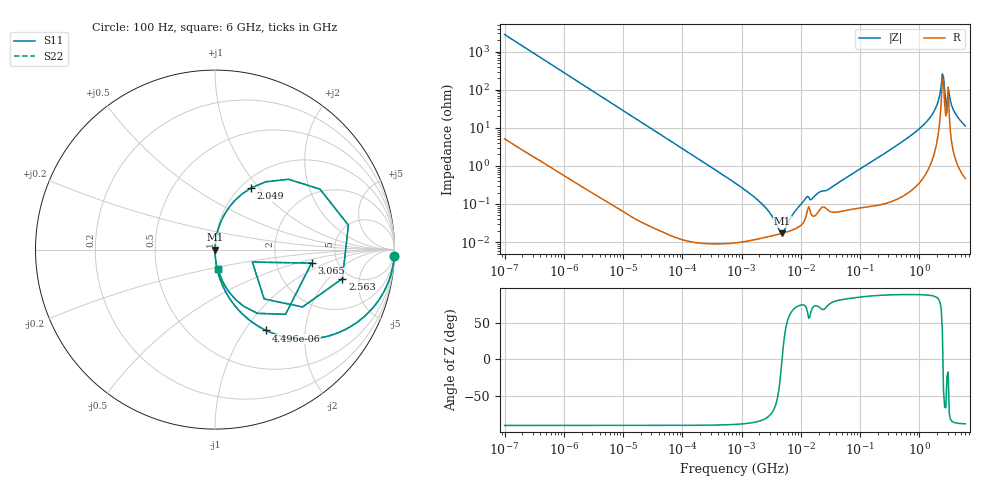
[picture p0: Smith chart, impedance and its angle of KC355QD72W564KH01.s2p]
!Murata Part Number: KC355QD72W564KH01
!These Parameters are Measured in Series Mode Connection
!Data Generated on Mar 13, 2026
!  o--ll--o
!Port1  Port2
!  o------o
!Operation Temp=25[degC], DC Bias Voltage=0[V]
!Freq. Start=100[Hz] Stop=6[GHz] 401[Steps]
# Hz S RI R 50
!Freq.(Hz) S11(Real) S11(Imag) S21(Real) S21(Imag) S12(Real) S12(Imag) S22(Real) S22(Imag)
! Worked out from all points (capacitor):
!   401 points, 100 Hz to 6 GHz, reference 50 ohm
!   read as one part in series: C = 563 nF near 109 Hz
!   lowest |Z| = 17 mohm at 4.857 MHz (marker M1)
!   series resonance near 4.826 MHz, so ESL is about 1.9 nH
!   S11 on the Smith chart (normalised r, x): 100 Hz: 1, -56; 4.496 kHz: 1.00, -1.26; 2.049 GHz: 1.11, +0.91; 2.563 GHz: 4.27, -2.93; 3.065 GHz: 3.22, -0.69; 6 GHz: 1.01, -0.22
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100  0.9987 -0.0354  0.00132 0.0354  0.00132 0.0354  0.9987 -0.0354
717  0.9393 -0.2378  0.0607 0.2378  0.0607 0.2378  0.9393 -0.2378
2008  0.6655 -0.4708  0.3345 0.4708  0.3345 0.4708  0.6655 -0.4708
4496  0.2853 -0.4505  0.7147 0.4505  0.7147 0.4505  0.2853 -0.4505
10527  0.0684 -0.2513  0.9316 0.2513  0.9316 0.2513  0.0684 -0.2513
40335  0.00515 -0.0702  0.9948 0.0702  0.9948 0.0702  0.00515 -0.0702
774597  0.000107 -0.00356  0.9999 0.00356  0.9999 0.00356  0.000107 -0.00356
2372521  0.000131 -0.00089  0.9999 0.00089  0.9999 0.00089  0.000131 -0.00089
4856642  0.00017 7.4e-06  0.9998 -7.4e-06  0.9998 -7.4e-06  0.00017 7.4e-06
1.189169e7  0.000409 0.00129  0.9996 -0.00129  0.9996 -0.00129  0.000409 0.00129
1.555665e7  0.000492 0.00129  0.9995 -0.00129  0.9995 -0.00129  0.000492 0.00129
3.124326e8  0.00176 0.0256  0.9982 -0.0256  0.9982 -0.0256  0.00176 0.0256
1.144649e9  0.0173 0.1116  0.9827 -0.1116  0.9827 -0.1116  0.0173 0.1116
1.712697e9  0.0712 0.2251  0.9288 -0.2251  0.9288 -0.2251  0.0712 0.2251
2.048624e9  0.2023 0.3443  0.7977 -0.3443  0.7977 -0.3443  0.2023 0.3443
2.240541e9  0.4091 0.3919  0.5909 -0.3919  0.5909 -0.3919  0.4091 0.3919
2.450438e9  0.7433 0.136  0.2567 -0.136  0.2567 -0.136  0.7433 0.136
2.562649e9  0.7103 -0.1612  0.2897 0.1612  0.2897 0.1612  0.7103 -0.1612
3.065283e9  0.5379 -0.0752  0.4621 0.0752  0.4621 0.0752  0.5379 -0.0752
3.352442e9  0.2368 -0.3552  0.7632 0.3552  0.7632 0.3552  0.2368 -0.3552
4.009986e9  0.07 -0.2241  0.93 0.2241  0.93 0.2241  0.07 -0.2241
6e9  0.0169 -0.1097  0.9831 0.1097  0.9831 0.1097  0.0169 -0.1097
